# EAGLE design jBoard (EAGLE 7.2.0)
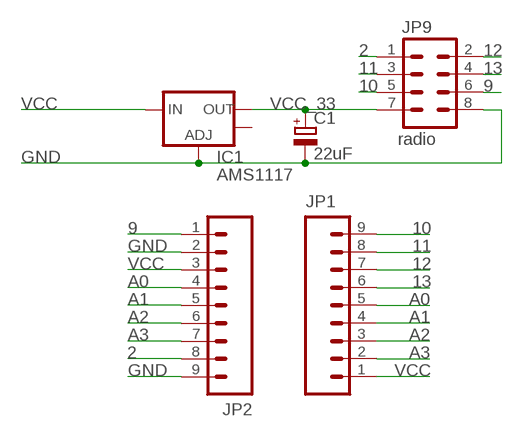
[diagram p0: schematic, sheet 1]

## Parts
C1  22uF  CPOL-EUE2.5-5  [E2,5-5]
IC1  AMS1117  V_REG_LM1117SOT223  [SOT223]
JP1  M09  [1X09]
JP2  M09  [1X09]
JP9  radio  M04X2  [2X4]

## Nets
2: JP2.8 JP9.1
9: JP2.1 JP9.6
10: JP1.9 JP9.5
11: JP1.8 JP9.3
12: JP1.7 JP9.2
13: JP1.6 JP9.4
A0: JP1.5 JP2.4
A1: JP1.4 JP2.5
A2: JP1.3 JP2.6
A3: JP1.2 JP2.7
GND: C1.- IC1.1(ADJ) JP2.2 JP2.9 JP9.8
VCC: IC1.3(IN) JP1.1 JP2.3
VCC_33: C1.+ IC1.2(OUT) JP9.7
Unconnected: IC1.4(OUT)

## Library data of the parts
C1 = rcl:CPOL-EU: POLARIZED CAPACITOR, European symbol
IC1 = SparkFun-PowerIC:V_REG_LM1117: Voltage Regulator LM1117 Standard adjustable voltage regulator but in SMD form. Spark Fun Electronics SKU : COM-00595; PROD_ID: VREG-08170
JP1 JP2 = SparkFun-Connectors:M09: Header 9 Standard 9-pin 0.1" header. Use with straight break away headers (SKU : PRT-00116), right angle break away headers (PRT-00553), swiss pins (PRT-00743), machine pins (PRT-00117), and female headers (PRT-00115).
JP9 = SparkFun-Connectors:M04X2: .1" header, two rows of four.

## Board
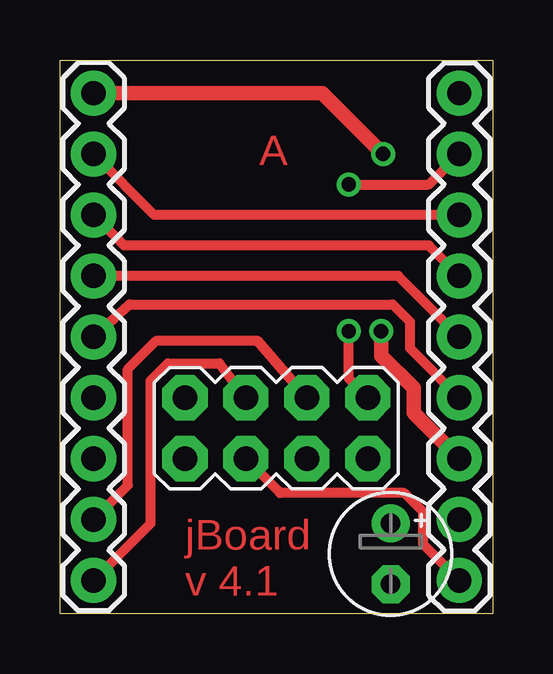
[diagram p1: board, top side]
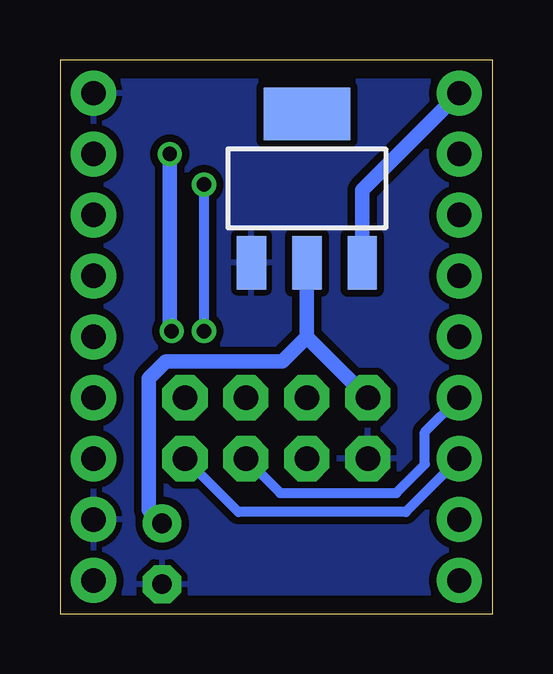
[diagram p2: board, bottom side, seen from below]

Size 18.03 x 23.1 mm. Coordinates in mm from the lower left corner, seen from the top.
Outline: 18.03,23.1 18.03,0 0,0 0,23.1 18.03,23.1
Copper layers (1*16): Top 0.035mm / dielectric 1.5mm / Bottom 0.035mm
Design rules "default *": minimum track width 10mil, minimum drill 24mil, track to track 12mil, track to pad 10mil, pad to pad 12mil, via to via 12mil, smd to smd 8mil, copper to edge 30mil, drill to drill 8mil, minimum pad ring 10mil, minimum via ring 8mil, stop-mask expansion 4mil, vias tented up to drill 0mil, thermal gap 10mil

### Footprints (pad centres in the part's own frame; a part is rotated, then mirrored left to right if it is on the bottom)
E2,5-5 = drill 0.813 pad 1.6: + -1.27,0 | drill 0.813 pad 1.6 octagon: - 1.27,0
SOT223 = smd 1.219 x 2.235: 1 -2.311,-3.099; 2 0,-3.099; 3 2.311,-3.099 | smd 3.6 x 2.2: 4 0,3.099
1X09 = drill 1.016 pad 1.88: 1 0,0; 2 2.54,0; 3 5.08,0; 4 7.62,0; 5 10.16,0; 6 12.7,0; 7 15.24,0; 8 17.78,0; 9 20.32,0
2X4 = drill 1.016 pad 1.88 octagon: 1 -3.81,-1.27; 2 -3.81,1.27; 3 -1.27,-1.27; 4 -1.27,1.27; 5 1.27,-1.27; 6 1.27,1.27; 7 3.81,-1.27; 8 3.81,1.27

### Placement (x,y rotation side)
C1  13.78,2.51 270 top
IC1  7.75,17.75 0 bottom
JP1  1.4,21.72 270 top
JP2  16.64,1.4 90 top
JP9  9.02,7.75 180 top

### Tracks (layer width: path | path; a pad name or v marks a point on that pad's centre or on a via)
2  (via drill 0.6)
  Top 0.406: JP9.1 12.03,9.81 v12.03,11.79 | v12.03,17.91 15.37,17.91 JP2.8
  Bottom 0.406: v12.03,11.79 v12.03,17.91
9
  Top 0.406: JP9.6 9.18,5.05 14.34,5.05 15.13,4.25 15.13,2.9 JP2.1
10
  Top 0.406: JP9.5 6.64,10.45 4.49,10.45 3.78,9.73 3.78,3.78 JP1.9
11
  Top 0.406: JP1.8 2.83,5.37 2.83,10.21 4.02,11.4 8.22,11.4 JP9.3
12
  Bottom 0.406: JP1.7 3.62,4.25 10.61,4.25 JP9.2
13
  Bottom 0.406: JP1.6 2.83,7.59 2.83,6.24 4.02,5.05 8.86,5.05 JP9.4
A0
  Top 0.406: JP1.5 2.9,12.91 13.86,12.91 14.57,12.19 14.57,11.08 JP2.4
A1
  Top 0.406: JP1.4 14.1,14.1 JP2.5
A2
  Top 0.406: JP1.3 2.67,15.37 15.37,15.37 JP2.6
A3
  Top 0.406: JP1.2 3.94,16.64 JP2.7
GND
  pour Bottom: -0.51,0.13 18.54,0.13 18.54,0.76 18.54,22.99 -0.51,22.99
VCC  (via drill 0.6)
  Top 0.61: JP2.3 14.73,8.38 14.73,9.41 13.38,10.76 v13.38,11.79 | JP1.1 10.92,21.72 v13.46,19.18
  Bottom 0.61: v13.38,11.79 13.46,11.88 v13.46,19.18 | JP1.1 5.44,17.68 IC1.3
VCC_33
  Bottom 0.61: JP9.7 7.75,11.56 | 7.75,11.56 IC1.2 | C1.+ 14.34,4.33 14.34,9.81 13.62,10.52 8.78,10.52 7.75,11.56

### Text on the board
Top: A | jBoard / v 4.1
